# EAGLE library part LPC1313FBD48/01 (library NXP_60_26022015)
32-bit ARM Cortex-M3 microcontroller; up to 32 kB flash and 8 kB SRAM; USB device The LPC1311/13/42/43 are ARM Cortex-M3 based microcontrollers for embedded applications featuring a high level of integration and low power consumption. The ARM Cortex-M3 is a next generation core that offers system enhancements such as enhanced debug features and a higher level of support block integration. The LPC1311/13/42/43 operate at CPU frequencies of up to 72 MHz. The ARM Cortex-M3 CPU incorporates a 3-stage pipeline and uses a Harvard architecture with separate local instruction and data buses as well as a third bus for peripherals. The ARM Cortex-M3 CPU also includes an internal prefetch unit that supports speculative branching. The peripheral complement of the LPC1311/13/42/43 includes up to 32 kB of flash memory, up to 8 kB of data memory, USB Device (LPC1342/43 only), one Fast-mode Plus I 2 C-bus interface, one UART, four general purpose timers, and up to 42 general purpose I/O pins. Remark: The LPC1311/13/42/43 series consists of the LPC1300 series (parts LPC1311/13/42/43) and the LPC1300L series (parts LPC1311/01 and LPC1313/01). The LPC1300L series features the following enhancements over the LPC1300 series: Power profiles with lower power consumption in Active and Sleep modes. Four levels for BOD forced reset. Second SSP controller (LPC1313FBD48/01 only). Windowed Watchdog Timer (WWDT). Internal pull-up resistors pull up pins to full VDD level. Programmable pseudo open-drain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
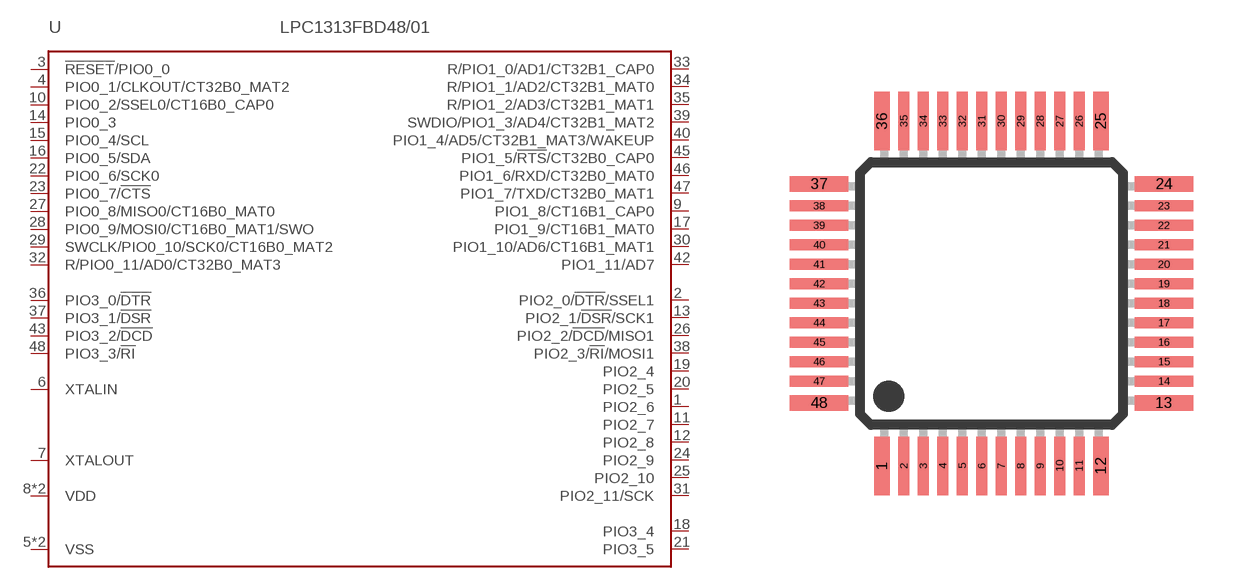
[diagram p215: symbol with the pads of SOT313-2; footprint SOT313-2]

Designator prefix U

## LPC1313FBD48/01 (ADC: 8; FLASH: 32kB; PWR_PROFILES: yes; SERIES: LPC1300L; SRAM: 8kB; SSP: 2; USB: -)  [SOT313-2]
1  PIO2_6
2  PIO2_0/!DTR!/SSEL1
3  !RESET!/PIO0_0
4  PIO0_1/CLKOUT/CT32B0_MAT2
5  VSS  pwr
6  XTALIN  in
7  XTALOUT  out
8  VDD  pwr
9  PIO1_8/CT16B1_CAP0
10  PIO0_2/SSEL0/CT16B0_CAP0
11  PIO2_7
12  PIO2_8
13  PIO2_1/!DSR!/SCK1
14  PIO0_3
15  PIO0_4/SCL
16  PIO0_5/SDA
17  PIO1_9/CT16B1_MAT0
18  PIO3_4
19  PIO2_4
20  PIO2_5
21  PIO3_5
22  PIO0_6/SCK0
23  PIO0_7/!CTS!
24  PIO2_9
25  PIO2_10
26  PIO2_2/!DCD!/MISO1
27  PIO0_8/MISO0/CT16B0_MAT0
28  PIO0_9/MOSI0/CT16B0_MAT1/SWO
29  SWCLK/PIO0_10/SCK0/CT16B0_MAT2
30  PIO1_10/AD6/CT16B1_MAT1
31  PIO2_11/SCK
32  R/PIO0_11/AD0/CT32B0_MAT3
33  R/PIO1_0/AD1/CT32B1_CAP0
34  R/PIO1_1/AD2/CT32B1_MAT0
35  R/PIO1_2/AD3/CT32B1_MAT1
36  PIO3_0/!DTR!
37  PIO3_1/!DSR!
38  PIO2_3/!RI!/MOSI1
39  SWDIO/PIO1_3/AD4/CT32B1_MAT2
40  PIO1_4/AD5/CT32B1_MAT3/WAKEUP
41  VSS  pwr
42  PIO1_11/AD7
43  PIO3_2/!DCD!
44  VDD  pwr
45  PIO1_5/!RTS!/CT32B0_CAP0
46  PIO1_6/RXD/CT32B0_MAT0
47  PIO1_7/TXD/CT32B0_MAT1
48  PIO3_3/!RI!

## Footprint SOT313-2 (pad centres in mm)
SOT313-2 LQFP48: plastic low profile quad flat package; 48 leads; body 7 x 7 x 1.4 mm JEDEC: MS-026 IEC: 136E05 Footprint according to NXP SOT313-2 specification, however the cornerpins are 0.4mm in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
smd 0.4 x 1.5: 1 -2.81,-4.425; 12 2.81,-4.425; 25 2.81,4.425; 36 -2.81,4.425
smd 0.28 x 1.5: 2 -2.25,-4.425; 3 -1.75,-4.425; 4 -1.25,-4.425; 5 -0.75,-4.425; 6 -0.25,-4.425; 7 0.25,-4.425; 8 0.75,-4.425; 9 1.25,-4.425; 10 1.75,-4.425; 11 2.25,-4.425; 26 2.25,4.425; 27 1.75,4.425; 28 1.25,4.425; 29 0.75,4.425; 30 0.25,4.425; 31 -0.25,4.425; 32 -0.75,4.425; 33 -1.25,4.425; 34 -1.75,4.425; 35 -2.25,4.425
smd 1.5 x 0.4: 13 4.425,-2.81; 24 4.425,2.81; 37 -4.425,2.81; 48 -4.425,-2.81
smd 1.5 x 0.28: 14 4.425,-2.25; 15 4.425,-1.75; 16 4.425,-1.25; 17 4.425,-0.75; 18 4.425,-0.25; 19 4.425,0.25; 20 4.425,0.75; 21 4.425,1.25; 22 4.425,1.75; 23 4.425,2.25; 38 -4.425,2.25; 39 -4.425,1.75; 40 -4.425,1.25; 41 -4.425,0.75; 42 -4.425,0.25; 43 -4.425,-0.25; 44 -4.425,-0.75; 45 -4.425,-1.25; 46 -4.425,-1.75; 47 -4.425,-2.25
